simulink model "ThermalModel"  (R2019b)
settings: Solver=ode45  StartTime=0.0  StopTime=10.0  RelTol=1e-3  EnableMultiTasking=on

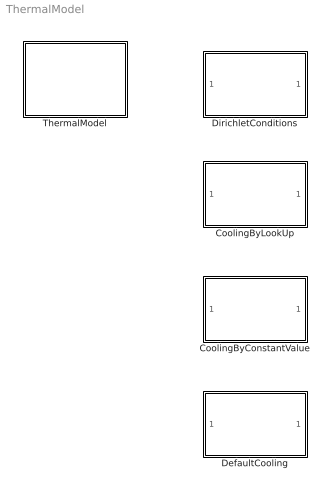
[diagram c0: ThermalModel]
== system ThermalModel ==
  CoolingByConstantValue : Subsystem
  CoolingByLookUp : Subsystem
  DefaultCooling : Subsystem
  DirichletConditions : Subsystem
  ThermalModel : Subsystem

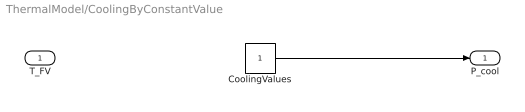
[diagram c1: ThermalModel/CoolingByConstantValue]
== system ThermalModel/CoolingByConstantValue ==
  T_FV : Inport
  CoolingValues : Constant
  P_cool : Outport  VectorParamsAs1DForOutWhenUnconnected=off
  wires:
  CoolingValues/1 -> P_cool/1

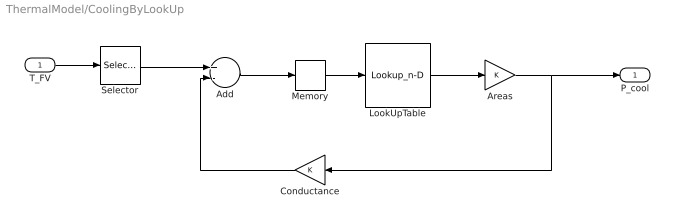
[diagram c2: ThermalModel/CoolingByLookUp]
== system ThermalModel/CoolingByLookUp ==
  T_FV : Inport
  Add : Sum  Inputs=+-
  Areas : Gain
  Conductance : Gain
  LookUpTable : Lookup_n-D  NumberOfTableDimensions=1  BreakpointsForDimension1=[-5:5]  Table=tanh([-5:5])  ExtrapMethod=Clip  RndMeth=Simplest
  Memory : Memory
  Selector : Selector  InputPortWidth=3  IndexOptions=Index vector (dialog)  Indices=[1 3]  OutputSizes=1
  P_cool : Outport  VectorParamsAs1DForOutWhenUnconnected=off
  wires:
  T_FV/1 -> Selector/1
  Selector/1 -> Add/1
  Add/1 -> Memory/1
  Conductance/1 -> Add/2
  Memory/1 -> LookUpTable/1
  LookUpTable/1 -> Areas/1
  Areas/1 -> Conductance/1, P_cool/1

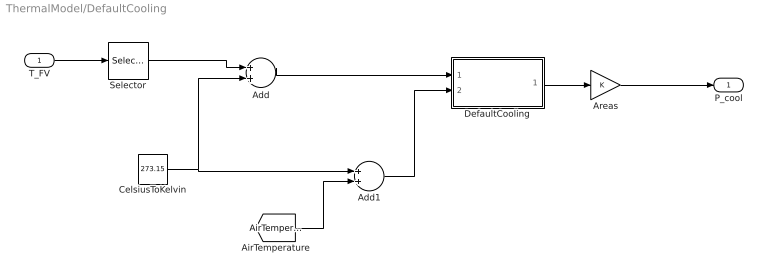
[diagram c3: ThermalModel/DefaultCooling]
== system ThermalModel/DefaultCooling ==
  T_FV : Inport
  Add : Sum
  Add1 : Sum
  Areas : Gain
  CelsiusToKelvin : Constant  Value=273.15
  DefaultCooling : MATLAB Function  TreatAsAtomicUnit=on
  Selector : Selector  InputPortWidth=3  IndexOptions=Index vector (dialog)  Indices=[1 3]  OutputSizes=1
  P_cool : Outport  VectorParamsAs1DForOutWhenUnconnected=off
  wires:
  T_FV/1 -> Selector/1
  Selector/1 -> Add/1
  Add/1 -> DefaultCooling/1(u)
  DefaultCooling/1(y) -> Areas/1
  Areas/1 -> P_cool/1
  CelsiusToKelvin/1 -> Add1/1, Add/2
  Add1/1 -> DefaultCooling/2(airTemperature)
  [AirTemperature] -> Add1/2

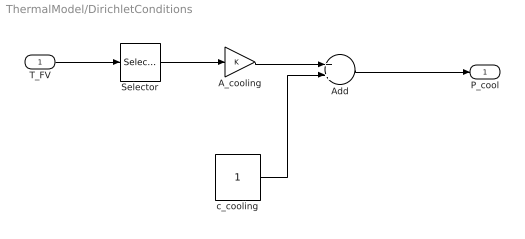
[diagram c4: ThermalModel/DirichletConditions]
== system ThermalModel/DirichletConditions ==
  T_FV : Inport
  A_cooling : Gain
  Add : Sum
  Selector : Selector  InputPortWidth=3  IndexOptions=Index vector (dialog)  Indices=[1 3]  OutputSizes=1
  c_cooling : Constant
  P_cool : Outport  VectorParamsAs1DForOutWhenUnconnected=off
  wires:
  T_FV/1 -> Selector/1
  c_cooling/1 -> Add/2
  Add/1 -> P_cool/1
  Selector/1 -> A_cooling/1
  A_cooling/1 -> Add/1

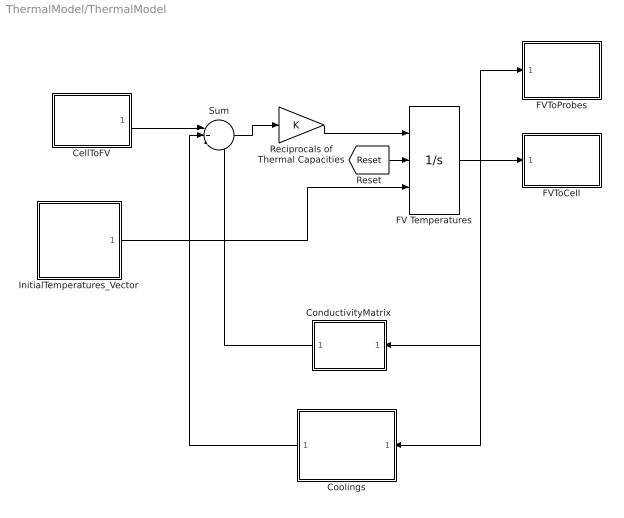
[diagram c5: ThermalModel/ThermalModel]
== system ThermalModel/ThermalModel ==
  CellToFV : Subsystem
  ConductivityMatrix : MATLAB Function  TreatAsAtomicUnit=on
  Coolings : Subsystem
  FV Temperatures : Integrator  ExternalReset=rising  InitialConditionSource=external
  FVToCell : Subsystem
  FVToProbes : Subsystem
  InitialTemperatures_Vector : Subsystem
  Reciprocals of Thermal Capacities : Gain
  Sum : Sum  Inputs=|+-+
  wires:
  Sum/1 -> Reciprocals of Thermal Capacities/1
  Reciprocals of Thermal Capacities/1 -> FV Temperatures/1
  FV Temperatures/1 -> FVToProbes/1(FVTemperatures), ConductivityMatrix/1(u), Coolings/1(T_FV), FVToCell/1(T_FV)
  Coolings/1(P_FV) -> Sum/2
  CellToFV/1(P_FV) -> Sum/1
  ConductivityMatrix/1(y) -> Sum/3
  [Reset] -> FV Temperatures/2
  InitialTemperatures_Vector/1(InitialTemperatures) -> FV Temperatures/3

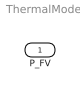
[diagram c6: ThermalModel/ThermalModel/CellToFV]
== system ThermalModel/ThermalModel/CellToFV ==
  P_FV : Outport  VectorParamsAs1DForOutWhenUnconnected=off

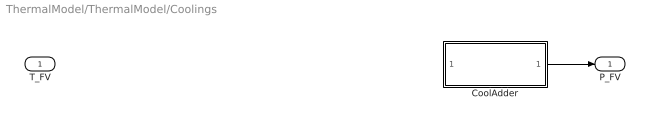
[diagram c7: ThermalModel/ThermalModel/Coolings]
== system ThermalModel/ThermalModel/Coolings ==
  T_FV : Inport
  CoolAdder : Subsystem
  P_FV : Outport  VectorParamsAs1DForOutWhenUnconnected=off
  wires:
  CoolAdder/1(P_FV) -> P_FV/1

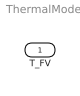
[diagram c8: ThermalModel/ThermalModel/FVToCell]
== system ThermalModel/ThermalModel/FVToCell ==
  T_FV : Inport

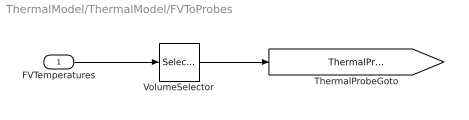
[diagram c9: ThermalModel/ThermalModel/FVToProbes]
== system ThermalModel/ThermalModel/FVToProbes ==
  FVTemperatures : Inport
  VolumeSelector : Selector  InputPortWidth=3  IndexOptions=Index vector (dialog)  Indices=[1 3]  OutputSizes=1
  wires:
  FVTemperatures/1 -> VolumeSelector/1
  VolumeSelector/1 -> [ThermalProbeTemperatures]

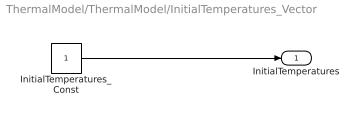
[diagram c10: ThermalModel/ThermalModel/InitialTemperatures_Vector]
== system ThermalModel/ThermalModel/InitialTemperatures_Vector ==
  InitialTemperatures_Const : Constant
  InitialTemperatures : Outport
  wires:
  InitialTemperatures_Const/1 -> InitialTemperatures/1

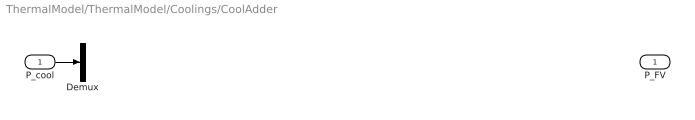
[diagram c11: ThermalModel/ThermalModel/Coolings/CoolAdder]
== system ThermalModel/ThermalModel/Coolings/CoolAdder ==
  P_cool : Inport
  Demux : Demux  Outputs=2
  P_FV : Outport  VectorParamsAs1DForOutWhenUnconnected=off
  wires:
  P_cool/1 -> Demux/1

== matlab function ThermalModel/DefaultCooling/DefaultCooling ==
function y = fcn(u, airTemperature)
    
y = DefaultCooling(u, airTemperature);

end

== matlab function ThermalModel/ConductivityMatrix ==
function y = fcn(u)
    y = ConductivityMatrix(u);
end
